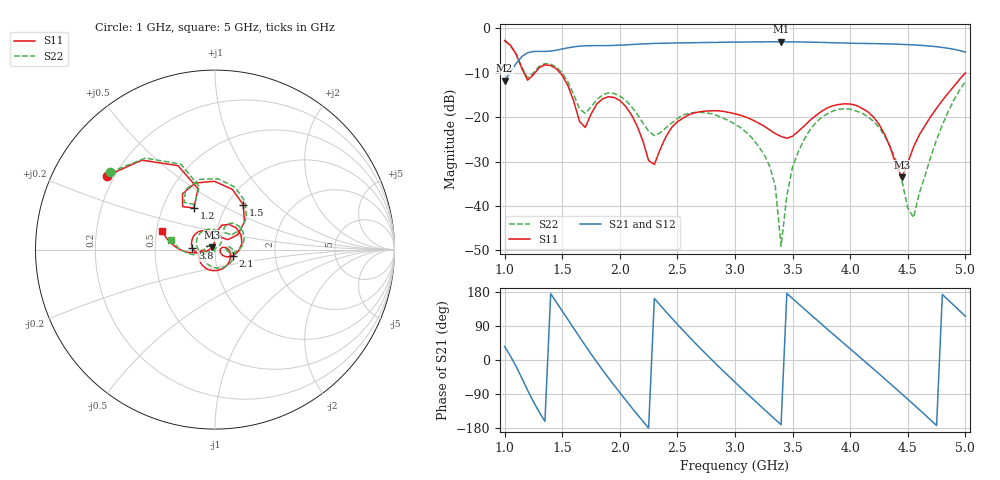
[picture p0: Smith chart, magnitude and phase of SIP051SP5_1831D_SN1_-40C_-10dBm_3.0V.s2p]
# GHz  S  dB  R  50
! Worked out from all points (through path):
!   81 points, 1 GHz to 5 GHz, reference 50 ohm
!   highest |S21| = -3.05 dB at 3.4 GHz (marker M1); lowest = -11.8 dB at 1 GHz (marker M2)
!   lowest |S11| = -33.5 dB at 4.45 GHz (marker M3), VSWR 1.04, Z = 48.4 + j1.26 ohm
!   |S11| at or under -10 dB: 1.168 GHz to 1.265 GHz (97.08 MHz wide, 7.98 % of centre); 1.48 GHz to end of sweep
!   |S22| runs from -49.1 to -2.8 dB; largest |S21 - S12| = 0.0018
!   S11 on the Smith chart (normalised r, x): 1 GHz: 0.17, +0.30; 1.2 GHz: 0.72, +0.36; 1.5 GHz: 1.18, +0.65; 2.1 GHz: 1.22, -0.08; 3.8 GHz: 0.78, +0.01; 5 GHz: 0.53, +0.12
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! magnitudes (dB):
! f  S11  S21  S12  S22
! 1 GHz  -2.7  -11.8  -11.8  -2.8
! 1.2 GHz  -11.7  -5.5  -5.5  -11.2
! 1.5 GHz  -10.6  -4.7  -4.7  -10.1
! 1.7 GHz  -22.3  -3.9  -4.0  -19.2
! 1.9 GHz  -15.4  -3.9  -3.9  -14.5
! 2.1 GHz  -19.4  -3.7  -3.7  -17.6
! 2.25 GHz  -29.8  -3.5  -3.5  -23.2
! 2.35 GHz  -27.3  -3.4  -3.4  -23.5
! 2.6 GHz  -19.5  -3.3  -3.3  -19.1
! 3 GHz  -19.3  -3.1  -3.1  -21.6
! 3.3 GHz  -22.9  -3.1  -3.1  -31.0
! 3.35 GHz  -23.7  -3.1  -3.1  -35.6
! 3.4 GHz  -24.4  -3.0  -3.0  -49.1
! 3.5 GHz  -24.3  -3.1  -3.1  -31.2
! 3.7 GHz  -19.7  -3.2  -3.2  -21.3
! 3.8 GHz  -17.9  -3.2  -3.2  -19.3
! 4.15 GHz  -18.7  -3.4  -3.4  -19.9
! 4.35 GHz  -27.0  -3.5  -3.6  -26.7
! 4.45 GHz  -33.5  -3.6  -3.6  -34.5
! 4.55 GHz  -26.7  -3.7  -3.8  -42.6
! 4.75 GHz  -18.0  -4.2  -4.2  -25.1
! 5 GHz  -10.1  -5.4  -5.4  -12.0
